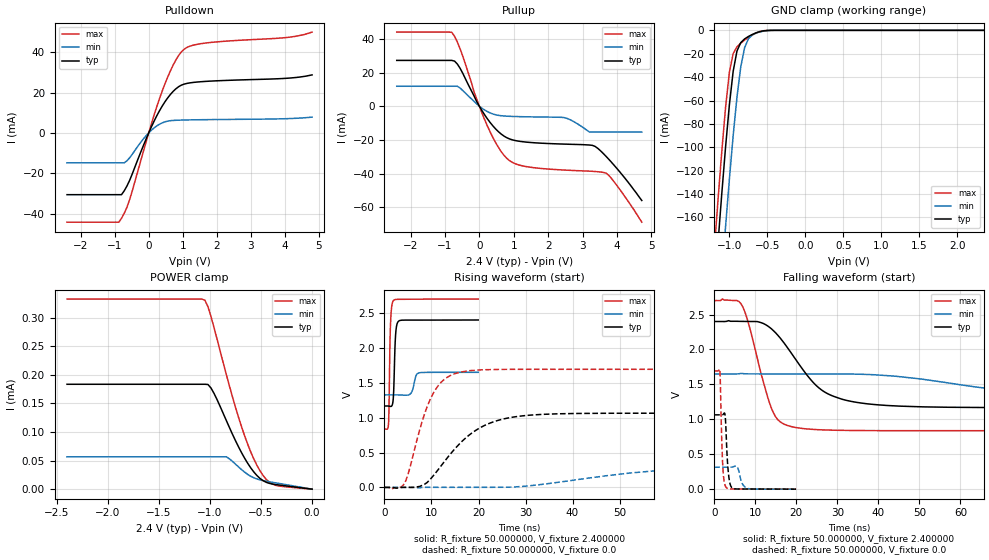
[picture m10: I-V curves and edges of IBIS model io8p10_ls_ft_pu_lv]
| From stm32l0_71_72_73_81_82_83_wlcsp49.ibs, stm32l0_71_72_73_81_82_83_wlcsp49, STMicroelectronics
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|   Model io8p10_ls_ft_pu_lv
[Model]  io8p10_ls_ft_pu_lv
Model_type I/O
Polarity   Non-Inverting
Enable   Active-Low
Vinl =   0.720000V
Vinh =   1.680000V
Vmeas =  1.200000V
Cref =   50.000000pF
Rref =   100.000000M
Vref =   0.0V
C_comp   4.521100pF   4.438000pF   4.578000pF
[Temperature Range]   25.000000   0.105000k   -40.000000
[Pullup Reference]   2.400000V   1.650000V   2.700000V
[Pulldown Reference]   0.0V   0.0V   0.0V
[POWER Clamp Reference]   2.400000V   1.650000V   2.700000V
[GND Clamp Reference]   0.0V   0.0V   0.0V
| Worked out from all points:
|   slope of the pulldown table from 0 to 0.36 V, typ, clamps not added: 29.5 ohm
|   slope of the pullup table from 0 to 0.36 V, typ, clamps not added: 33.2 ohm
|   GND clamp passes 1 mA (typ) near -0.59 V on its own axis
|   rising waveform, R_fixture 50.000000, V_fixture 2.400000: 20-80 % time 359ps typ, 684ps min, 299ps max; typ from 1.17 V to 2.4 V
|   rising waveform, R_fixture 50.000000, V_fixture 0.0: 20-80 % time 9.3ns typ, 24.6ns min, 4.8ns max; typ from 0.001 V to 1.06 V
|   falling waveform, R_fixture 50.000000, V_fixture 2.400000: 20-80 % time 10.1ns typ, 28ns min, 5.05ns max; typ from 2.4 V to 1.17 V
|   falling waveform, R_fixture 50.000000, V_fixture 0.0: 20-80 % time 624ps typ, 991ps min, 519ps max; typ from 1.06 V to 0.001 V
[Pulldown]
|Voltage   I(typ)   I(min)   I(max)
-2.4V     -30.64mA   -14.84mA   -44.29mA
-880mV    -30.64mA   -14.84mA   -44.29mA
-800mV    -30.64mA   -14.84mA   -42.37mA
-720mV    -28.74mA   -14.84mA   -39.91mA
-560mV    -23.52mA   -12.34mA   -33.09mA
0V        -765nA     -61nA      -2.526uA
400mV     13.38mA    4.998mA    20.91mA
720mV     20.62mA    6.178mA    33.69mA
1.04V     24.19mA    6.384mA    41.49mA
1.6V      25.46mA    6.544mA    44.42mA
4V        27.03mA    7.028mA    47.23mA
4.8V      28.76mA    7.817mA    49.99mA
[Pullup]
|Voltage   I(typ)   I(min)   I(max)
-2.4V     27.23mA    11.87mA    44.05mA
-800mV    27.23mA    11.87mA    43.87mA
-560mV    22.57mA    10.83mA    34.16mA
-160mV    6.379mA    3.022mA    8.973mA
240mV     -7.653mA   -3.251mA   -12mA
560mV     -15.22mA   -5.43mA    -24.63mA
800mV     -18.73mA   -5.908mA   -31mA
1.28V     -21.13mA   -6.236mA   -35.54mA
2.48V     -22.51mA   -6.818mA   -37.93mA
3.36V     -23.83mA   -15.36mA   -38.77mA
3.76V     -31.49mA   -15.36mA   -41.07mA
4.72V     -56mA      -15.36mA   -68.89mA
[GND_clamp]
|Voltage   I(typ)   I(min)   I(max)
-2.4V     -1.379A    -1.445A    -1.35A
-1.2V     -225.9mA   -297.5mA   -189.2mA
-1.15V    -182mA     -253.1mA   -145.3mA
-1.1V     -139.6mA   -209.7mA   -103.5mA
-1.05V    -99.61mA   -167.6mA   -65.7mA
-1V       -63.67mA   -127.3mA   -35.89mA
-950mV    -35mA      -89.93mA   -19.87mA
-900mV    -17.67mA   -57.01mA   -14.12mA
-850mV    -10.49mA   -31.18mA   -11mA
-750mV    -5.288mA   -7.322mA   -5.997mA
-450mV    -33.57uA   -87.56uA   -14.35uA
2.35V     0A         0A         0A
[POWER_clamp]
|Voltage   I(typ)   I(min)   I(max)
-2.4V     183.5uA    56.67uA    332.6uA
-1.05V    183.5uA    56.67uA    330.7uA
-1.02V    183.2uA    56.67uA    319.4uA
-960mV    167.5uA    56.67uA    282.5uA
-840mV    120.2uA    56.67uA    200.6uA
-750mV    84.84uA    43.79uA    143.2uA
-690mV    63.63uA    34.11uA    108.8uA
-600mV    37.11uA    22.45uA    64.86uA
-510mV    18.78uA    16.35uA    32.08uA
-450mV    12.09uA    14.02uA    17.37uA
-360mV    8.168uA    11.12uA    6.844uA
0V        0A         0A         0A
[Ramp]
| variable   typ   min   max
dV/dt_r  0.63803/9.28799n   0.18818/24.69217n   1.01576/4.78667n
dV/dt_f  0.73962/10.09489n   0.19398/27.99375n   1.11752/5.04222n
R_load = 50.000000
[Rising Waveform]
R_fixture= 50.000000
V_fixture= 2.400000
V_fixture_min= 1.650000
V_fixture_max= 2.700000
|time   V(typ)   V(min)   V(max)
0s        1.167V     1.327V     837.5mV
840.8ps   1.167V     1.327V     896.2mV
961ps     1.165V     1.327V     1.149V
1.281ns   1.162V     1.327V     2.338V
1.882ns   1.287V     1.327V     2.675V
2.362ns   2.184V     1.327V     2.694V
3.003ns   2.382V     1.326V     2.696V
5.606ns   2.398V     1.348V     2.697V
7.447ns   2.398V     1.643V     2.698V
19.94ns   2.4V       1.65V      2.7V
[Rising Waveform]
R_fixture= 50.000000
V_fixture= 0.0
V_fixture_min= 0.0
V_fixture_max= 0.0
|time   V(typ)   V(min)   V(max)
0s        1.051mV    1.39mV     741.8uV
4.505ns   1.702mV    1.474mV    92.62mV
8.509ns   45.73mV    1.916mV    1.051V
11.01ns   220.5mV    2.319mV    1.42V
14.01ns   479mV      2.315mV    1.604V
18.02ns   751.2mV    2.332mV    1.673V
25.03ns   977.1mV    3.277mV    1.692V
37.04ns   1.056V     75.12mV    1.693V
85.59ns   1.064V     306.4mV    1.693V
249.2ns   1.064V     315mV      1.693V
[Falling Waveform]
R_fixture= 50.000000
V_fixture= 2.400000
V_fixture_min= 1.650000
V_fixture_max= 2.700000
|time   V(typ)   V(min)   V(max)
0s        2.4V       1.65V      2.7V
6.507ns   2.402V     1.656V     2.656V
8.008ns   2.401V     1.651V     2.443V
14.51ns   2.264V     1.65V      1.083V
17.02ns   2.093V     1.65V      931.6mV
22.02ns   1.678V     1.65V      865.4mV
29.03ns   1.331V     1.65V      844.7mV
45.05ns   1.189V     1.611V     837.9mV
95.6ns    1.167V     1.352V     837.5mV
249.2ns   1.167V     1.327V     837.5mV
[Falling Waveform]
R_fixture= 50.000000
V_fixture= 0.0
V_fixture_min= 0.0
V_fixture_max= 0.0
|time   V(typ)   V(min)   V(max)
0s        1.064V     315mV      1.693V
1.361ns   1.064V     315mV      1.704V
2.082ns   1.066V     315mV      344.7mV
2.603ns   1.077V     315mV      65.61mV
2.883ns   837mV      314.9mV    28.53mV
3.443ns   241mV      314.6mV    7.879mV
4.324ns   21.66mV    317.5mV    4.052mV
5.606ns   3.472mV    321.8mV    3.829mV
8.208ns   2.963mV    10.07mV    2.335mV
19.94ns   1.051mV    1.39mV     741.8uV
